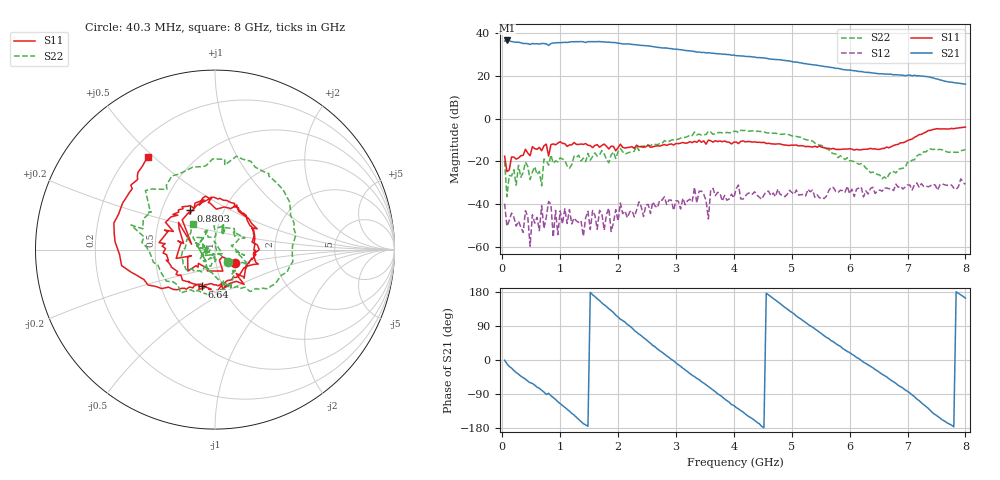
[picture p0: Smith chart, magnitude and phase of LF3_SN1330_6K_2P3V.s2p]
! VC=2.3V I=17.45mA
# HZ S DB R 50.00
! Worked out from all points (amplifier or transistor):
!   200 points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, 40.3 MHz to 8 GHz, reference 50 ohm
!   highest |S21| = 36.5 dB at 80.3 MHz (marker M1)
!   |S21| within 3 dB of that: start of sweep to 2.627 GHz
!   unconditionally stable (mu >= 1): start of sweep to 3.302 GHz; 3.748 GHz to 4.022 GHz; 4.1 GHz to end of sweep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
!   at 1.36 GHz: K = 1.93, MAG = 36.3 dB, |S12| = -47.7 dB
!   at 4.04 GHz: K = 0.92, MSG = 31.1 dB, |S12| = -32.7 dB
!   at 8 GHz: K = 1.68, MAG = 18.6 dB, |S12| = -30.7 dB
!   S11 on the Smith chart (normalised r, x): 40.3 MHz: 1.23, -0.18; 880.3 MHz: 0.70, +0.32; 6.64 GHz: 0.80, -0.34; 8 GHz: 0.28, +0.48
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4.02985e7  -17.54 -33.5  36.23 -0.5  -39.68 138.2  -19.83 -43.7
8.0297e7  -24.73 -44.2  36.49 -9.7  -50.25 -1.0  -36.44 -47.4
3.20288e8  -17.35 -133.9  35.42 -42.6  -50.64 -165.7  -27.33 171.7
8.80267e8  -11.78 122.2  35.33 -99.3  -55.33 -163.4  -20.87 133.4
1.160256e9  -12.29 77.7  35.73 -135.0  -42.45 31.1  -23.21 90.7
1.400248e9  -12.01 35.4  35.85 -168.1  -54.89 87.2  -18.46 63.4
1.680237e9  -13.34 -6.8  35.99 156.8  -42.82 66.3  -16.95 43.4
2.040224e9  -11.94 -50.0  35.09 107.6  -39.37 -46.4  -13.89 -25.2
2.320213e9  -12.39 -88.4  34.50 73.2  -42.70 -85.2  -12.63 -68.7
2.720198e9  -12.82 -128.5  33.18 24.5  -37.92 -53.9  -11.64 -114.6
3.000188e9  -11.62 -158.3  32.43 -7.6  -38.25 -109.1  -9.71 -157.5
3.400172e9  -10.06 172.9  31.11 -51.8  -33.93 -130.5  -7.24 156.8
3.760159e9  -10.42 132.8  30.27 -92.9  -34.76 -162.3  -6.45 120.6
4.040148e9  -10.93 102.5  29.39 -125.4  -32.72 -169.7  -5.92 83.9
4.560129e9  -11.62 65.8  28.18 176.2  -34.01 153.3  -6.59 25.9
4.960114e9  -12.54 33.9  26.90 129.9  -33.46 102.1  -7.52 -17.4
5.360099e9  -13.31 -0.7  25.14 86.7  -33.36 59.2  -10.44 -50.3
6.000075e9  -14.05 -47.6  22.71 19.7  -35.05 27.0  -19.63 -116.0
6.640051e9  -13.25 -109.3  20.80 -44.4  -32.42 -37.4  -28.09 -95.0
6.68005e9  -13.63 -112.6  20.76 -49.6  -32.72 -37.1  -26.01 -95.0
7.440021e9  -5.06 175.5  19.03 -140.3  -30.58 -100.1  -14.41 -154.4
8e9  -3.92 126.1  16.09 163.2  -30.70 -155.1  -14.41 130.3
